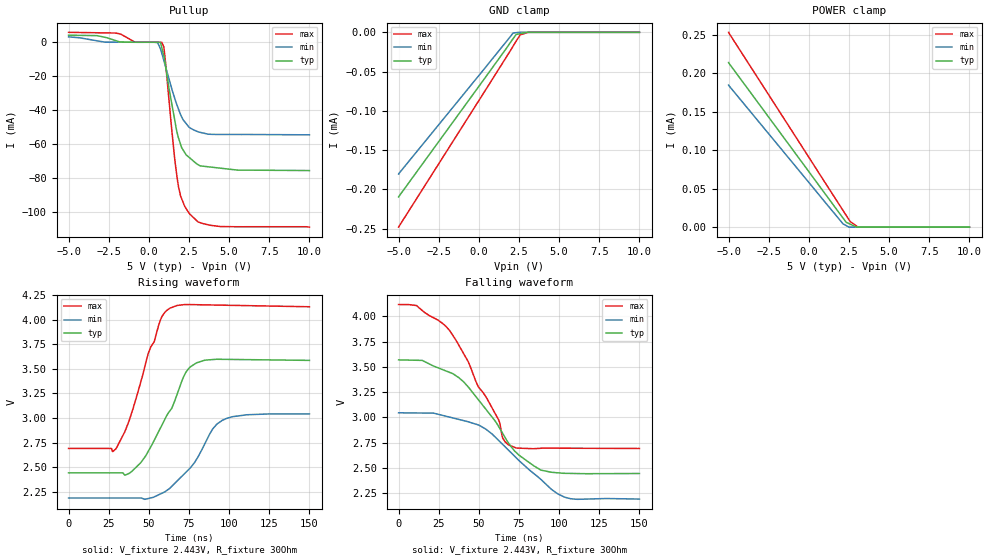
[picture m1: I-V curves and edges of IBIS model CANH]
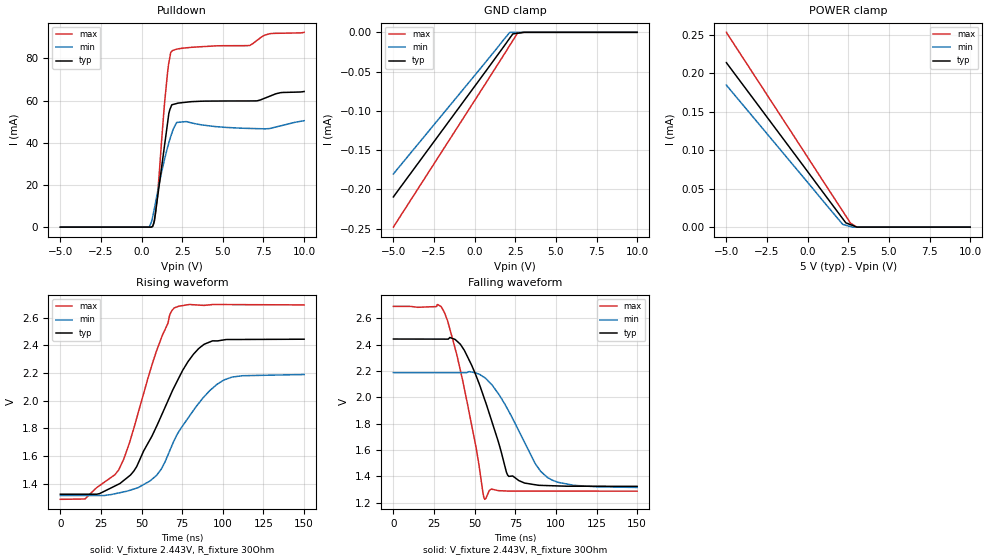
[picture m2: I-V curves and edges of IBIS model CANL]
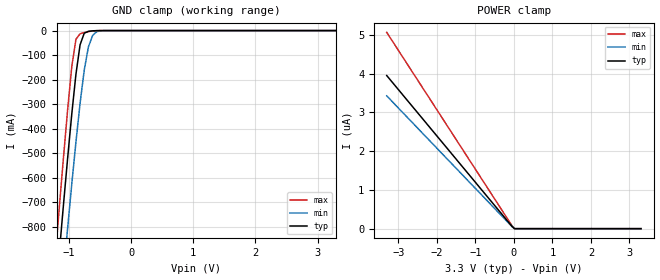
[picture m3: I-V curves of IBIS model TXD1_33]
| IBIS file created by Layout Workbench Version 22.1.4.12161.401368   004
| Cadence Design Systems, Inc. 2011
[IBIS ver]   4.2
[File name]  isow1050v.ibs
[File Rev]   1.5
[Date]   06 15, 2026
[Source]   Model built from TISPICED simulations at:
   Texas Instruments Incorporated.
   Analog-eLab, HPA 12500 TI Blvd
   Dallas, TX -75243
   For Support e-mail: elab_ibis@list.ti.com
[Notes]   This product is designed as an aid for customers of Texas Instruments.
   No warranties, either expressed or implied, with respect to this third party software (if any)
   or with respect to its fitness for any particular purpose is claimed by Texas Instruments or
   the author. The software (if any) is provided solely on an "as is" basis. The entire risk as to
   its quality and performance is with the customer
[Disclaimer]  This product is designed as an aid for customers of Texas Instruments. No warranties, either expressed or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
[Copyright] (C)Copyright 2025 Texas Instruments Incorporated. All rights reserved.
|   Component ISOW1050V
[Component] ISOW1050V
[Manufacturer] Texas Instruments Incorporated
[Package]   |16-pin SOIC DWE package
|   typ   min   max
R_pkg   0.04817   0.03432   0.09530
L_pkg   2.4595nH   1.6904nH   4.7034nH
C_pkg   0.847pF   0.428pF   1.397pF
[Pin]  signal_name   model_name   R_pin   L_pin   C_pin
1   VDD1   POWER   0.03455  3.39778n  0.89677p
2   GND1   GND   0.03432  3.12613n  0.84706p
3   TXD   TXD1   0.04265  1.85523n  0.57831p
4   NC   NC   0.04783  1.99000n  0.60148p
5   RXD   RXD1   0.06147  2.13194n  0.42769p
6   NC   NC   0.04783  1.99000n  0.60148p
7   VDDL   POWER   0.04783  1.99000n  0.60148p
8   GND1   GND   0.03740  4.70338n  1.39696p
9   GND2   GND   0.03763  4.61305n  1.39587p
10   GND2   GND   0.04703  2.01514n  0.58483p
11   VISOIN   POWER   0.07132  2.45946n  0.43321p
12   CANL   CANL   0.03943  1.70546n  0.55709p
13   CANH   CANH   0.07288  2.39260n  0.48001p
14   NC   NC   0.04783  1.99000n  0.60148p
15   GND2   GND   0.04817  4.23145n  0.93567p
16   VISOOUT   POWER   0.04790  4.51154n  0.99405p
[Model Selector] RXD1
RXD_25   RXD Output model for 2.25V - 2.75V
RXD_33   RXD Output model for 3.0V - 3.6V
RXD_5   RXD Output model for 4.5V - 5.5V
[Model Selector] TXD1
TXD1_25   TXD Input Model for 2.25V - 2.75V
TXD1_33   TXD Input model for 3.0V - 3.6V
TXD1_5   TXD Input model for 4.5V - 5.5V
| Models and submodels in the file (8): CANH (I/O_open_source), CANL (I/O_open_drain), TXD1_33 (Input), TXD1_5 (Input), TXD1_25 (Input), RXD_33 (3-state), RXD_5 (3-state), RXD_25 (3-state)
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[Model]   CANH
Model_type   I/O_open_source
Polarity   Inverting
Enable   Active-Low
Vinl = 0.5
Vinh = 0.9
Vmeas = 3
Vref = 2.443
Cref = 2pF
Rref = 30
|   typ   min   max
C_comp   12.2e-12   11.49e-12   12.57e-12
[Voltage Range]   5   4.5   5.5
[Temperature Range]   25   150   -55
[Pullup Reference]   5   4.5   5.5
[Pulldown Reference]   0   0   0
[Power Clamp Reference]   5   4.5   5.5
[GND Clamp Reference]   0   0   0
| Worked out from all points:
|   slope of the pullup table from 0 to 0.75 V, typ, clamps not added: 727 ohm
|   falling waveform, V_fixture 2.443V, R_fixture 30Ohm: 20-80 % time 31.2ns typ, 35.1ns min, 29.3ns max; typ from 3.57 V to 2.44 V
|   rising waveform, V_fixture 2.443V, R_fixture 30Ohm: 20-80 % time 20.2ns typ, 21.6ns min, 16.6ns max; typ from 2.44 V to 3.59 V
[GND Clamp]
|   Voltage   I(typ)   I(min)   I(max)
-5V       -209.7uA   -180.5uA   -248.2uA
2.128V    -8.187uA   -910.9nA   -17.7uA
2.322V    -2.722uA   -432nA     -11.25uA
2.569V    -1.686uA   0A         -3.295uA
3.064V    0A         0A         0A
10V       0A         0A         0A
[Pullup]
|   Voltage   I(typ)   I(min)   I(max)
-5V       4.168mA    3.187mA    5.861mA
-2.061V   962.1uA    55.5uA     5.435mA
-861.1mV  8.134uA    7.958uA    128.5uA
482.5mV   3.073uA    -99.63uA   3.64uA
797.2mV   -2.85mA    -6.239mA   -7.214uA
930.8mV   -8.028mA   -10.68mA   -2.658mA
1.594V    -45.06mA   -32.61mA   -67.39mA
1.848V    -56.59mA   -39.51mA   -85.28mA
2.229V    -65.02mA   -46.88mA   -96.72mA
3.064V    -72.18mA   -52.81mA   -106mA
4.442V    -74.24mA   -54.38mA   -108.7mA
10V       -75.66mA   -54.59mA   -109mA
[POWER Clamp]
|   Voltage   I(typ)   I(min)   I(max)
-5V       213.6uA    184.5uA    252.9uA
2.128V    11.78uA    4.269uA    21.63uA
2.322V    6.298uA    2.025uA    15.35uA
2.569V    3.9uA      0A         7.37uA
3.064V    0A         0A         0A
10V       0A         0A         0A
[Ramp]
R_load = 30
|   typ   min   max
dV/dt_r   0.685442/2.00542e-08   0.512592/2.14191e-08   0.863536/1.66139e-08
dV/dt_f   0.674704/3.11586e-08   0.512317/3.5057e-08   0.855212/2.92131e-08
[Falling Waveform]
V_fixture = 2.443V
V_fixture_min = 2.188V
V_fixture_max = 2.691V
R_fixture = 30Ohm
C_fixture = 0F
|   Time   V(typ)   V(min)   V(max)
0s        3.569V     3.045V     4.117V
11.28ns   3.565V     3.043V     4.106V
31.67ns   3.445V     3.002V     3.861V
50.06ns   3.167V     2.923V     3.294V
62.3ns    2.909V     2.772V     2.975V
64.87ns   2.84V      2.731V     2.793V
68.51ns   2.745V     2.674V     2.726V
88.48ns   2.479V     2.388V     2.694V
103.4ns   2.446V     2.21V      2.694V
150ns     2.444V     2.191V     2.691V
[Rising Waveform]
V_fixture = 2.443V
V_fixture_min = 2.188V
V_fixture_max = 2.691V
R_fixture = 30Ohm
C_fixture = 0F
|   Time   V(typ)   V(min)   V(max)
0s        2.443V     2.188V     2.691V
29.42ns   2.443V     2.188V     2.686V
37.65ns   2.437V     2.188V     2.97V
45.02ns   2.548V     2.188V     3.371V
57.13ns   2.897V     2.228V     3.994V
62.96ns   3.071V     2.285V     4.115V
75.77ns   3.519V     2.493V     4.153V
89.67ns   3.594V     2.888V     4.148V
95.81ns   3.596V     2.978V     4.147V
150ns     3.586V     3.042V     4.13V
|   CANL Model
[Model]   CANL
Model_type   I/O_open_drain
Polarity   Non-Inverting
Enable   Active-Low
Vinl = 0.5
Vinh = 0.9
Vmeas = 2
Vref = 2.443
Cref = 2pF
Rref = 30
|   typ   min   max
C_comp   11.96e-12   11.44e-12   12.21e-12
[Voltage Range]   5   4.5   5.5
[Temperature Range]   25   150   -55
[Pullup Reference]   5   4.5   5.5
[Pulldown Reference]   0   0   0
[Power Clamp Reference]   5   4.5   5.5
[GND Clamp Reference]   0   0   0
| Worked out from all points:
|   slope of the pulldown table from 0 to 0.75 V, typ, clamps not added: 373 ohm
|   falling waveform, V_fixture 2.443V, R_fixture 30Ohm: 20-80 % time 18.1ns typ, 22.3ns min, 14.4ns max; typ from 2.44 V to 1.32 V
|   rising waveform, V_fixture 2.443V, R_fixture 30Ohm: 20-80 % time 27.4ns typ, 26.3ns min, 22.2ns max; typ from 1.32 V to 2.44 V
[Pulldown]
|   Voltage   I(typ)   I(min)   I(max)
-5V       30fA       -53.22pA   460fA
252.8mV   4.719uA    -3.121uA   -1.871uA
647.3mV   194.8uA    3.573mA    145.6uA
782.7mV   2.825mA    8.677mA    2.945mA
979mV     13.95mA    16.53mA    15.09mA
1.407V    38.49mA    32.05mA    58.45mA
1.6V      49.55mA    37.9mA     73.56mA
1.894V    58.11mA    45.29mA    83.7mA
2.755V    59.27mA    50.08mA    85.07mA
6.669V    59.86mA    46.81mA    86.22mA
7.601V    61.23mA    46.63mA    91.14mA
10V       64.34mA    50.49mA    92.41mA
[GND Clamp]
|   Voltage   I(typ)   I(min)   I(max)
-5V       -209.7uA   -180.5uA   -248.2uA
2.155V    -7.531uA   -153.4nA   -16.77uA
2.349V    -2.037uA   -103.9nA   -10.51uA
2.638V    -1.181uA   -29.97nA   -1.117uA
3.037V    0A         0A         0A
10V       0A         0A         0A
[POWER Clamp]
|   Voltage   I(typ)   I(min)   I(max)
-5V       213.6uA    184.5uA    252.9uA
2.155V    11.02uA    3.595uA    20.77uA
2.349V    5.558uA    2.436uA    14.52uA
2.638V    3.222uA    702.3nA    5.157uA
3.031V    53.18nA    0A         0A
10V       0A         0A         0A
[Ramp]
R_load = 30
|   typ   min   max
dV/dt_r   0.671493/2.72876e-08   0.524178/2.61335e-08   0.842197/2.20483e-08
dV/dt_f   0.671494/1.80697e-08   0.523421/2.22127e-08   0.842202/1.44627e-08
[Falling Waveform]
V_fixture = 2.443V
V_fixture_min = 2.188V
V_fixture_max = 2.691V
R_fixture = 30Ohm
C_fixture = 0F
|   Time   V(typ)   V(min)   V(max)
0s        2.443V     2.188V     2.691V
27.22ns   2.443V     2.188V     2.706V
31.4ns    2.443V     2.188V     2.646V
41.22ns   2.404V     2.188V     2.205V
56.2ns    1.983V     2.15V      1.226V
60.2ns    1.832V     2.101V     1.303V
71.01ns   1.4V       1.894V     1.288V
87.3ns    1.336V     1.497V     1.288V
94.67ns   1.33V      1.393V     1.288V
150ns     1.324V     1.316V     1.288V
[Rising Waveform]
V_fixture = 2.443V
V_fixture_min = 2.188V
V_fixture_max = 2.691V
R_fixture = 30Ohm
C_fixture = 0F
|   Time   V(typ)   V(min)   V(max)
0s        1.324V     1.315V     1.288V
15.16ns   1.324V     1.315V     1.29V
35.89ns   1.397V     1.334V     1.5V
45.28ns   1.493V     1.362V     1.803V
59.14ns   1.813V     1.46V      2.358V
67.49ns   2.033V     1.643V     2.626V
70ns      2.097V     1.711V     2.668V
85.22ns   2.377V     1.982V     2.69V
100.8ns   2.439V     2.15V      2.694V
150ns     2.444V     2.189V     2.691V
|   TXD1_33 Model
[Model]   TXD1_33
Model_type Input
Polarity   Non-Inverting
Enable   Active-High
Vinl =  0.990V
Vinh =  2.310V
C_comp   1.300pF   1.100pF   1.500pF
[Model Spec]
Vinh   2.310V   2.079V   2.541V
Vinl   0.990V   0.891V   1.089V
[Temperature Range]   27.000   0.150k   -55.000
[Voltage Range]   3.300V   3.000V   3.600V
[POWER Clamp Reference]   3.300V   3.000V   3.600V
[GND Clamp Reference]   0.0V   0.0V   0.0V
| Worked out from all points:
|   GND clamp passes 1 mA (typ) near -0.62 V on its own axis
[GND_clamp]
|Voltage   I(typ)   I(min)   I(max)
-3.3V     -6.511A    -6.3A      -6.742A
-1.223V   -1.108A    -1.374A    -932.4mA
-1.156V   -908.9mA   -1.182A    -724.2mA
-1.089V   -712.9mA   -993.1mA   -520.4mA
-1.022V   -522.3mA   -807.7mA   -324.9mA
-955mV    -341.3mA   -627.5mA   -147.8mA
-888mV    -178.8mA   -455.4mA   -35.62mA
-821mV    -57.82mA   -296.5mA   -13.04mA
-754mV    -10.68mA   -161mA     -8.05mA
-687mV    -2.941mA   -66.52mA   -4.244mA
-553mV    -287.9uA   -4.329mA   -378.7uA
3.3V      0A         0A         -460.3nA
[POWER_clamp]
|Voltage   I(typ)   I(min)   I(max)
-3.3V     3.95uA     3.427uA    5.064uA
-50mV     59.91nA    53.72nA    76.8nA
17mV      0A         0A         0A
3.3V      0A         0A         0A
